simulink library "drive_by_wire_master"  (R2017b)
settings: Solver=ode1  StartTime=0.0  StopTime=Inf  FixedStep=0.001  RelTol=1e-3  EnableMultiTasking=on
PostLoadFcn:
  | , if any(exist('dsrtsu_mdlpostloadfcn', 'file') == [2, 3, 6]), try dsrtsu_mdlpostloadfcn('Execute', bdroot); catch fprintf('Error in PostLoadFcn (dsrtsu_mdlpostloadfcn) for model "%s":\n %s\n', bdroot, lasterr); end, end,
libraries: rtican x1

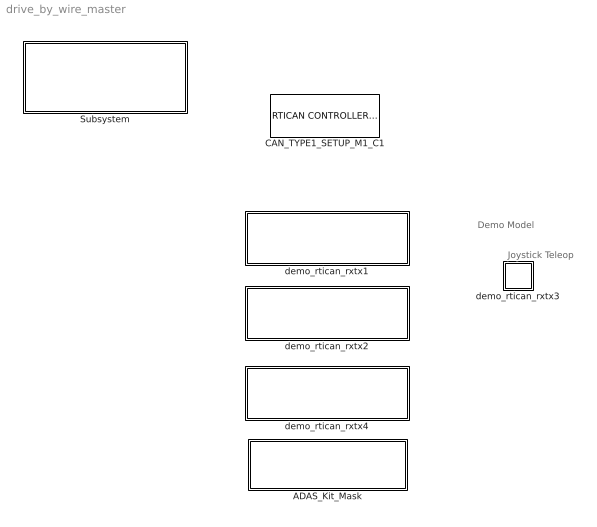
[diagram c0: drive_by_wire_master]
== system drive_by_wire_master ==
  note: Demo Model
  note: Joystick Teleop
  ADAS_Kit_Mask : Subsystem
  CAN_TYPE1_SETUP_M1_C1 : rtican/RTICAN CONTROLLER SETUP   Reserved1=[]  Reserved2=[]  Reserved3=[]  Reserved4=[]  AcceptanceMask=[]  ArbitrationField=[]  Parameters=[]  SFcnRTICANSettings=[]  MS_Struct=[]  BoardTypeNo=[]  BoardNo=[]  ChannelNo=[]  DialogFcn=[]  UnitName=[]  Revision=[]  UnitValues=[]  DSProperties=struct('RTI',struct('Version',uint32(12),'BlockType',struct('isSLSource',uint8(0),'isSLSink',uint8(0),'isHWSource',uint8(0),'isHWSink',uint8(0),'isSetup',uint8(1),'isInline',uint8(1),'isNonInline',uint8(0),'isInterrupt',uint8(0),'isChannelwise',uint8(0)),'IOBoardType','RTICAN','UnitType','NON_MESSAGE','Identifier','MASTER','DialogType','ML','BlockSet','RTICAN','SlaveProcessor','CAN'))  RTIBlockInterface=struct('InputPortsWidth',int32(0),'InputPortsActive',0,'OutputPortsWidth',int32(0),'OutputPortsActive',0,'DialogFcn','rtican_master_setup_gui','BlockDisplay',{{['CAN CONTROLLER\n SETUP'],'center'}},'IconTransparency','on','InitLevel',3,'IWork',{{{'',uint32(2)}}},'BlockName',struct('Token',{{'CAN_TYPE','_SETUP_M','_C'}},'BlockParam',{{'BoardTypeNo','BoardNo','ChannelNo'}}),'ParameterTunableNames',{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  RTIBlockParameters=struct('BoardTypeNo',{{1,'OFF',[]}},'BoardNo',{{1,'ON',[1 16]}},'ChannelNo',{{1,'ON',[1 2]}},'AcceptanceMask',{{0,'OFF',[]}},'ArbitrationField',{{0,'OFF',[]}},'Parameters',{{struct('Config',struct('Baudrate',500,'SampleMode',1,'UsedParamSet',1,'validSettings',1,'isBTRvalues',0,'Advanced',struct('Baudrate',{500,500,500},'Frequency',{24000000,36000000,64000000},'Settings',{struct('SMPL',0,'BRP',0,'N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  RTISFcnParameters=struct('SFcnRTICANSettings','struct','SFcnRTICCPSettings','struct','SFcnRTIXCPSettings','struct','AcceptanceMask','int32','ArbitrationField','int32','TLCFileName','char')  RTIBlockParaDefault=struct('BoardTypeNo',4302,'BoardNo',1,'ChannelNo',1,'AcceptanceMask',0,'ArbitrationField',0,'Parameters',struct('Config',struct('Baudrate',500,'SampleMode',1,'UsedParamSet',1,'validSettings',1,'isBTRvalues',0,'Advanced',struct('Frequency',16000000,'BTR0',64,'BTR1',28,'Settings',struct('SMPL',0,'BRP',0,'NBT',16,'TSEG1',12,'TSEG2',1,'SJW',1,'SP',87))),'configType',1,'Options',struct('DataFileSelecte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
  Subsystem : Subsystem
  demo_rtican_rxtx1 : Subsystem  mask(CAN_TYPE1){}
  demo_rtican_rxtx2 : Subsystem  mask(CAN_TYPE1){}
  demo_rtican_rxtx3 : Subsystem  mask(CAN_TYPE1){}
  demo_rtican_rxtx4 : Subsystem  mask(CAN_TYPE1){}

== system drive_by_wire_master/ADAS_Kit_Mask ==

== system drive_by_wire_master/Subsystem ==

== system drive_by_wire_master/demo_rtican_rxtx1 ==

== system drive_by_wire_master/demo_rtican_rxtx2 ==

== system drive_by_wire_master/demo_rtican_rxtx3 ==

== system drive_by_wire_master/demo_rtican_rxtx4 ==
